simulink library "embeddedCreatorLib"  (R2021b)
settings: Solver=VariableStepAuto  StartTime=0.0  StopTime=10.0  RelTol=1e-3
undefined symbols (not defined in the file or in its folder): B, based, C, classic, dsPic33, MCC, Microchip, PIC24, Sunday, U1, U2, Y1, Y2

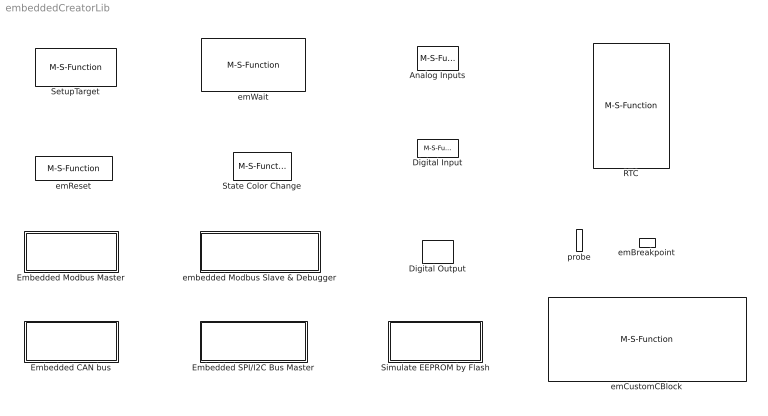
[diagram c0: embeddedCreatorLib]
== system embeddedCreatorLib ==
  Analog Inputs : M-S-Function  Tag=AnalogInputs  FunctionName=Ain2  Parameters=c_ADC_DeviceNo,c_AinQty,c_AChannelQty,c_AnalogOutFormat,c_Scale,c_Offset,c_SOC_Method,c_SAMSAMPLE,c_ADCTime,c_DMAChannelNo,c_sampleTime  mask(Analog Input){c_ADC_DeviceNo=1, c_AinQty=4, c_AChannelQty=3, c_AnalogOutFormat=16 bits signed interger Data, c_Scale=[2 5 4/9 5/77 ], c_Offset=[1 2 3 4], c_SOC_Method=Other Peripheral triggered SOC and ADC interrupt Enabled, c_SAMSAMPLE=on, c_ADCTime=100, c_DMAChannelNo=0, c_sampleTime=-1}
      mask prompts: c_ADC_DeviceNo "Peripheral Analog Device  Number:"; c_AinQty "Analog Inputs Qty:"; c_AChannelQty "Analog Channel or Core Qty:"; c_AnalogOutFormat "block output Data Format for Analog:"; c_Scale "Scale ( Value/bit):"; c_Offset "Offset (Raw Data when value is 0):"; c_SOC_Method "ADC start and handle method"; c_SAMSAMPLE "Simultaneously Sampling"; c_ADCTime "ADC minimum sampling time in ns"; c_DMAChannelNo "DMA Channel No:"; c_sampleTime "Sample time in sec (-1 for inherited):"
      mask help: Analog inputs
      mask init:
      | try
      | set_param(gcs,'Lock',"off");
      | set_param(gcbh,'MaskSelfModifiable',"on");
      | end
  Digital Input : M-S-Function  FunctionName=Din2  Parameters=c_Name_method,c_PortName,c_BitNo,c_DinAccessName,c_EnableFilter,c_Filter_method,c_filterQTY,c_initialV,c_sampleTime  mask(Digital Input){c_Name_method=By physical port name and bit number, c_PortName=B, c_BitNo=4, c_DinAccessName="PORTBbits.RB4", c_EnableFilter=on, c_Filter_method=Continuous sample multiple times in one sample period, c_filterQTY=12, c_initialV=0, c_sampleTime=-1}
      mask prompts: c_Name_method "How to specify Digital Input"; c_PortName "Port Name:"; c_BitNo "Port Bit number:"; c_DinAccessName "C Variable/Func Name"; c_EnableFilter "Enable Filter"; c_Filter_method "Filter Selection"; c_filterQTY "Sample Qty used in digital filter:"; c_initialV "Initial Input Value:"; c_sampleTime "Sample time in sec (-1 for inherited):"
      mask help: Digital Input
      mask init:
      | try
      | set_param(gcs,'Lock',"off");
      | set_param(gcbh,'MaskSelfModifiable',"on");
      | end
  Digital Output : M-S-Function  FunctionName=Dout2  Parameters=c_Name_method,c_PortName,c_BitNo,c_DinAccessName,c_initialV,c_sampleTime  mask(Digital Output){c_Name_method=By physical port name and bit number, c_PortName=C, c_BitNo=3, c_DinAccessName="LATCbits.LATC3", c_initialV=1, c_sampleTime=-1}
      mask prompts: c_Name_method "How to specify Digital Output"; c_PortName "Port Name:"; c_BitNo "Port Bit number:"; c_DinAccessName "C Variable/Func Name"; c_initialV "Initial Output Value:"; c_sampleTime "Sample time in sec (-1 for inherited):"
      mask help: Digital Output
      mask init:
      | try
      | set_param(gcs,'Lock',"off");
      | set_param(gcbh,'MaskSelfModifiable',"on");
      | end
  Embedded CAN bus : Subsystem
  Embedded Modbus Master : Subsystem
  Embedded SPI/I2C Bus Master : Subsystem
  RTC : M-S-Function  Tag=RTCC  FunctionName=RTC2  Parameters=c_PowerOn_resetClock,c_Year,c_Month,c_Day,c_Week,c_hour,c_Minute,c_Seconds,c_sampleTime  mask(RTC){c_PowerOn_resetClock=on, c_Year=2024, c_Month=10, c_Day=27, c_Week=Sunday, c_hour=0, c_Minute=0, c_Seconds=0, c_sampleTime=-1}
      mask prompts: c_PowerOn_resetClock "Set Clock initial Value from parameters when Power on"; c_Year "Year:"; c_Month "Month:"; c_Day "Day:"; c_Week "Week:"; c_hour "Hour:"; c_Minute "Minutes:"; c_Seconds "Seconds:"; c_sampleTime "Sample time in sec (-1 for inherited):"
      mask help: This is embedded "Real Time Clock" You can set "year/monrh/day/week/hour/minute/second" in parameters. When input port "En" is false, the clock can be set from other input ports. If both parameter and input port set the same item, input port has higher priority. For example, Input port " Yr" sets "2023" when "En"= false, but parameter "Yr" sets "2028". System will take "2023". When input port "En" is true, "RTC" will update clock automatically, and you can know "Year/Month/..../Sec" from output port. If parameter "Set Clock intial Value from parameters when Power on" checked, RTC will get init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
      mask init:
      | try
      |     set_param(gcs,'Lock',"off");
      |     set_param(gcbh,'MaskSelfModifiable',"on");
      | end
  SetupTarget : M-S-Function  Tag=SetupTarget  Priority=0  FunctionName=setupTarget2  Parameters=c_platform,c_debug  mask(Embedded Target platform selection){c_platform=Microchip PIC24/dsPic33 based on MCC classic, c_debug=on}
      mask prompts: c_platform "Target Platform"; c_debug "Debug Enabled for Simulink"
      mask help: We support multiple embedded target platforms (Bare Metal Microcontroller platform)
  Simulate EEPROM by Flash : Subsystem
  State Color Change : M-S-Function  FunctionName=ColorDisplay2  Parameters=g_tag,g_QTY  mask(Display Activated block){g_tag="State", g_QTY=2}
      mask prompts: g_tag "Tag name for All Action blocks which denote FSM's states"; g_QTY "Action Sub-Block QTY:"
      mask help: These blocks are for displaying activated block in Green color. It is used for State machine which is implemented by "switch case" or "if-else" blocks. The states are conditional "Action Subsystem" blocks. Inside each "Action Subsystem" block, you must put this "Color Display" Block in order to make State visibility.
  emBreakpoint : M-S-Function  Tag=emBreakpoint  FunctionName=emBreakpoint2  Parameters=c_enableBK, c_times4break, c_continue,c_ObjID,c_serverID,c_UartNo,c_StartAddr4FirstBK,c_firstEnter  mask{c_enableBK=on, c_times4break=1, c_continue=off, c_ObjID=-1, c_serverID=0, c_UartNo=0, c_StartAddr4FirstBK=0, c_firstEnter=off}
      mask prompts: c_enableBK "Enable Breakpoint"; c_times4break "How many executing times to create one break ?"; c_continue "Continue Run (Now it is no use)"; c_ObjID "Obj_ID"; c_serverID "Debug Server ID"; c_UartNo "Debug Server uart"; c_StartAddr4FirstBK "Address of  First BK (0 based)"; c_firstEnter "First time enter this (change to exteral trigger by continur button)"
      mask init:
      | try
      | set_param(gcs,'Lock',"off");
      | set_param(gcbh,'MaskSelfModifiable',"on");
      | end
  emCustomCBlock : M-S-Function  Tag=emCustomBlock  FunctionName=emCustomCBlock2  Parameters=c_InputDataName, c_InputDataType, c_OutputDataName,c_OutputDataType,c_InputDataQty,c_InputType,c_OutputDataQty,c_OutputType,c_sampleTime, c_blockname  mask(embedded Custom C Code){c_InputDataName=[U1 U2], c_InputDataType=[uint16 uint32], c_OutputDataName=[Y1 Y2], c_OutputDataType=[uint16 uint16], c_InputDataQty=[1  1], c_InputType=[5  7], c_OutputDataQty=[1  1], c_OutputType=[5  5], c_sampleTime=-1, c_blockname=[]}
      mask prompts: c_InputDataName "Input Port Variable Name in C language"; c_InputDataType "Input Port data type"; c_OutputDataName "Output Port Variable Name in C language"; c_OutputDataType "Output Port data type"; c_InputDataQty "InputDataQTY"; c_InputType "InputDataType"; c_OutputDataQty "OutputDataQty"; c_OutputType "OutputDataType"; c_sampleTime "Sample time in sec (-1 for inherited):"; c_blockname "BlockNameWhenCompiled"
      mask help: This is for user to add C Code manually. Input/Output port name and data type can be set in parameters. And Input/Output port names are the same as C language variable names. User's Code has 2 parts. One part is Only running once for initialization. The other part is running peridically in your settings sample time. The position for the 1st part code you want to add is between comment "//Customized Initialization Code for Block: emCustomCBlock ------Start" and "//Customized Initialization Code for Block: emCustomCBlock ------End" The position for the 2nd part code you want to add is between co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
      mask init:
      | try
      |     set_param(gcs,'Lock',"off");
      |     set_param(gcbh,'MaskSelfModifiable',"on");
      | end
  emReset : M-S-Function  Tag=emReset  FunctionName=emReset2  Parameters=c_serverID, c_UartNo, c_StartAddr  mask(embedded Reset){c_serverID=1, c_UartNo=2, c_StartAddr=1}
      mask prompts: c_serverID "Debug Server ID"; c_UartNo "Debug Server uart"; c_StartAddr "Address of  Mine (1 based)"
      mask help: Reset Target Micro-controller.
      mask init:
      | try
      |     set_param(gcs,'Lock',"off");
      |     set_param(gcbh,'MaskSelfModifiable',"on");
      | end
  emWait : M-S-Function  Tag=emWait  FunctionName=emWait2  Parameters=c_hours,c_minutes,c_seconds,c_ms,c_ObjID,c_serverID,c_UartNo,c_sampleTime  mask(embedded Wait){c_hours=0, c_minutes=0, c_seconds=12, c_ms=2, c_ObjID=0, c_serverID=1, c_UartNo=0, c_sampleTime=-1}
      mask prompts: c_hours "How many hours to wait?"; c_minutes "How many minutes to wait?"; c_seconds "How many seconds to wait?"; c_ms "How many ms to wait?"; c_ObjID "Obj_ID"; c_serverID "Debug Server ID"; c_UartNo "Debug Server uart"; c_sampleTime "Sample time in sec (-1 for inherited):"
      mask help: This block will wait for some time (hours/minutes/seconds) in non-blocking way. When any of input ports "Min"/"Sec"/"0,1Sec" connected, the initial waiting time is decided by these input ports (unconnected part is 0). When input port "En" is false, waiting time will be initialized. Of cause, when power on, waiting time will be initialized too. When input port "En" is true, this block starts counting-down for delay time. When time is on, output port "On" will be true, and output ports "Hr"/"Min"/"Sec" will be 0 ( time left). Maximum delay time from parameters is 255 hours 59 minutes 59 seconds 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
      mask init:
      | try
      |     set_param(gcs,'Lock',"off");
      |     set_param(gcbh,'MaskSelfModifiable',"on");
      | end
  embedded Modbus Slave & Debugger : Subsystem
  probe : M-S-Function  Tag=emProbe  FunctionName=emProbe2  Parameters=c_ObjID,c_serverID,c_UartNo,c_StartAddr,c_ConstantDataSource  mask(embedded Probe){c_ObjID=-1, c_serverID=1, c_UartNo=4, c_StartAddr=[], c_ConstantDataSource=on}
      mask prompts: c_ObjID "Obj_ID"; c_serverID "Debug Server ID"; c_UartNo "Debug Server uart"; c_StartAddr "Address of  Mine (1 based)"; c_ConstantDataSource "Constant Source Data"
      mask help: Probe is used for watching Simulink Signal by connecting "Display" block
      mask init:
      | try
      |     set_param(gcs,'Lock',"off");
      |     set_param(gcbh,'MaskSelfModifiable',"on");
      | end

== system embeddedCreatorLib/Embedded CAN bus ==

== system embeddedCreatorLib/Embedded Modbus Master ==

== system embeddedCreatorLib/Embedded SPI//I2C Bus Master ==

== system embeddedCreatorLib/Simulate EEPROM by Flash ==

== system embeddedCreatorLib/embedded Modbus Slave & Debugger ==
